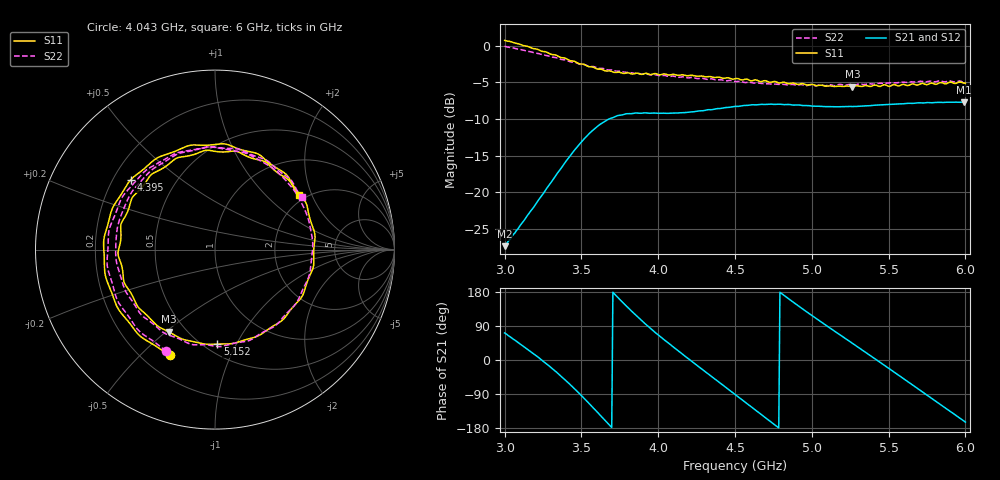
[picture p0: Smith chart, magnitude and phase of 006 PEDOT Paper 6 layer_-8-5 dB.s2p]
!  04/11/2025  19:26:33
! Ref Plane: 0.000 mm
# MHZ S MA R  50
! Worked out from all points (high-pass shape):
!   401 points, 3 GHz to 6 GHz, reference 50 ohm
!   highest |S21| = -7.70 dB at 5.992 GHz (marker M1); lowest = -27.4 dB at 3 GHz (marker M2)
!   |S21| within 3 dB of the highest: 3.624 GHz to end of sweep
!   lowest |S11| = -5.6 dB at 5.265 GHz (marker M3), VSWR 3.21, Z = 20.2 - j25.5 ohm
!   |S11| at or under -10 dB: nowhere
!   |S22| runs from -5.5 to -0.1 dB; largest |S21 - S12| = 0.0084
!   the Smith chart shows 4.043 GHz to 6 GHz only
!   S11 on the Smith chart (normalised r, x): 4.043 GHz: 0.31, -0.61; 4.395 GHz: 0.27, +0.34; 5.152 GHz: 0.58, -0.84; 6 GHz: 1.84, +1.60
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3000  1.086 -113.5  0.04283 71.5  0.0432 72.6  0.9917 -117.7
3142.5  0.993 -147.3  0.06795 30.4  0.06797 31.3  0.9202 -151.0
3270  0.9067 179.6  0.1048 -9.0  0.1049 -8.0  0.8595 175.5
3390  0.8245 143.0  0.1576 -50.8  0.1581 -50.3  0.801 138.0
3502.5  0.75 101.8  0.2218 -95.0  0.2222 -94.6  0.7446 96.5
3637.5  0.6857 45.3  0.2975 -152.4  0.2991 -151.9  0.7 40.1
3735  0.6588 1.5  0.3332 166.0  0.3338 166.9  0.6693 -2.0
3870  0.6472 -53.4  0.3465 112.2  0.349 113.2  0.6469 -56.5
4005  0.6339 -100.7  0.3455 64.8  0.3454 65.6  0.6248 -103.2
4042.5  0.6412 -113.2  0.3457 52.2  0.3484 52.9  0.6265 -115.6
4222.5  0.6272 -168.0  0.3533 -4.8  0.355 -4.1  0.6072 -171.4
4395  0.6097 140.2  0.3724 -58.3  0.3743 -57.3  0.585 134.9
4500  0.5951 107.4  0.385 -91.0  0.3874 -90.2  0.5692 101.8
4635  0.5843 65.6  0.3944 -132.7  0.3956 -132.2  0.5555 58.4
4762.5  0.5688 25.8  0.3975 -172.3  0.3978 -171.5  0.5468 18.0
5002.5  0.5438 -46.6  0.3871 116.9  0.3868 117.6  0.5396 -53.4
5152.5  0.5263 -88.6  0.3823 74.8  0.3824 75.5  0.5331 -96.1
5265  0.5253 -119.5  0.3844 43.9  0.3851 44.4  0.5399 -126.3
5505  0.5277 173.4  0.3973 -23.1  0.3992 -22.1  0.5573 167.6
5767.5  0.552 97.6  0.4086 -97.7  0.4104 -96.7  0.573 94.8
5992.5  0.5547 35.5  0.412 -161.5  0.4137 -160.8  0.5624 33.5
6000  0.555 33.0  0.4116 -163.8  0.4131 -163.1  0.5632 31.1
